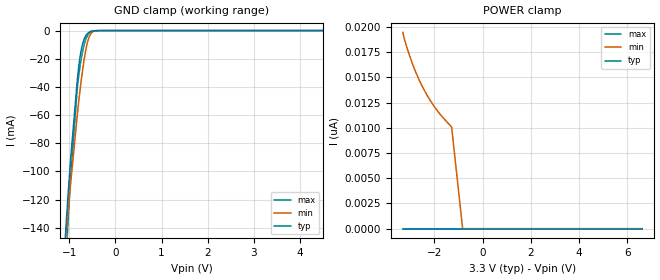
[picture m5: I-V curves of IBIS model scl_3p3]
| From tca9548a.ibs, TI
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|   scl_3p3 Model
[Model]   scl_3p3
Model_type   Input
Vinl = 0.99
Vinh = 2.31
|   typ   min   max
|   (nom PVT)   (fast PVT)   (slow PVT)
C_comp   6.033e-12   5.589e-12   6.668e-12
[Model spec]
|subparameter
Vinl   0.99   0.9   1.08
Vinh   2.31   2.1   2.52
|Where nom  PVT is Nominal Process, 3.3V, 27C
|   Fast PVT is Strong Process,  3.6V, -40C
|   Slow PVT is Weak Process,   3V, 125C
[Voltage Range]   3.3   3   3.6
|Junction Temperature
[Temperature Range]   27   125   -40
[Power Clamp Reference]   3.3   3   3.6
[GND Clamp Reference]   0   0   0
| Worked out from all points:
|   GND clamp passes 1 mA (typ) near -0.56 V on its own axis
[GND Clamp]
|   Voltage   I(typ)   I(min)   I(max)
-3.3V     -1.776A    -1.403A    -2.2A
-1.185V   -196.5mA   -192.5mA   -237.5mA
-1.047V   -125.6mA   -136.5mA   -147mA
-1.016V   -111.1mA   -124.8mA   -128.7mA
-974.4mV  -91.88mA   -109.2mA   -104.7mA
-825mV    -33.93mA   -58.78mA   -39.54mA
-771mV    -19.31mA   -43.02mA   -26.03mA
-711.6mV  -9.255mA   -27.71mA   -14.79mA
-620.4mV  -2.613mA   -10.08mA   -4.353mA
-541.2mV  -683.9uA   -2.553mA   -978.2uA
-260.7mV  -638.7nA   -3.821uA   -274.6nA
6.6V      0A         0A         0A
[POWER Clamp]
|   Voltage   I(typ)   I(min)   I(max)
-3.3V     0A         19.47nA    0A
-3.249V   0A         18.91nA    0A
-3.162V   0A         18.17nA    0A
-2.88V    0A         16.2nA     0A
-2.748V   0A         15.42nA    0A
-2.472V   0A         14nA       0A
-2.293V   0A         13.21nA    0A
-2.013V   0A         12.16nA    0A
-1.671V   0A         11.09nA    0A
-1.281V   0A         10.08nA    0A
-825mV    0A         0A         0A
6.6V      0A         0A         0A
